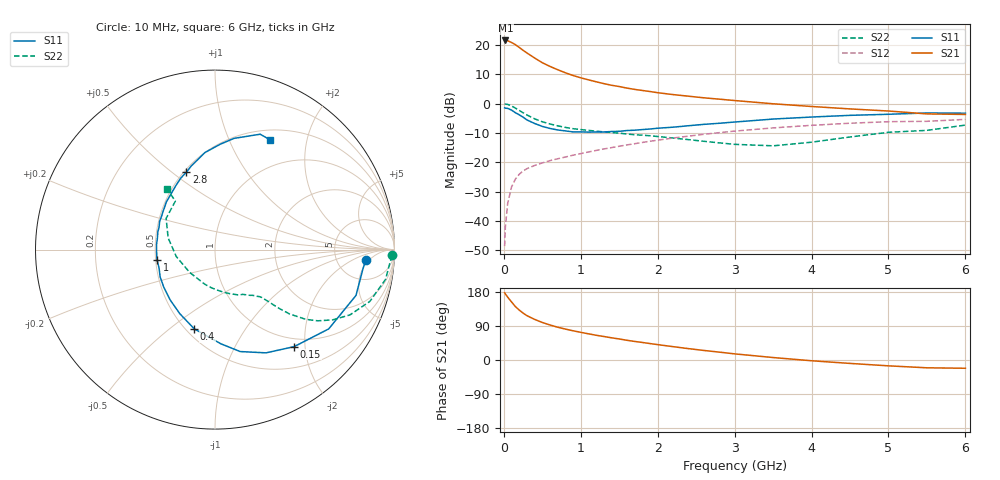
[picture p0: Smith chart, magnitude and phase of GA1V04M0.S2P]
! Infineon Technologies  Discrete & RF Semiconductors
! BF775
! Si NPN RF Bipolar Junction Transistor in SOT23
! VCE = 1 V  IC = 4 mA
! Common Emitter S-Parameters:  May  1996
# GHz  S  MA  R  50
!  f  S11  S21  S12  S22
! GHz  MAG  ANG  MAG  ANG  MAG  ANG  MAG  ANG
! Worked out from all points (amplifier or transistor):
!   36 points, 10 MHz to 6 GHz, reference 50 ohm
!   highest |S21| = 21.5 dB at 20 MHz (marker M1)
!   |S21| within 3 dB of that: start of sweep to 232.1 MHz
!   unconditionally stable (mu >= 1): 793.3 MHz to end of sweep
!   at 250 MHz: K = 0.44, MSG = 20.6 dB, |S12| = -23.0 dB
!   at 1.4 GHz: K = 1.17, MAG = 8.1 dB, |S12| = -15.0 dB
!   at 6 GHz: K = 1.04, MAG = -0.4 dB, |S12| = -5.4 dB
!   S11 on the Smith chart (normalised r, x): 10 MHz: 10, -4; 150 MHz: 0.85, -1.79; 400 MHz: 0.55, -0.61; 1 GHz: 0.51, -0.06; 2.8 GHz: 0.51, +0.56; 6 GHz: 0.62, +1.43
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0.01  0.8431 -3.8  11.81 177.4  0.0037 86.9  0.9891 -1.9
0.02  0.8318 -7.1  11.88 174.1  0.0079 85.2  0.9783 -4.0
0.05  0.826 -18.0  11.76 165.9  0.0198 79.5  0.9647 -9.9
0.1  0.7723 -34.9  10.98 153.3  0.0377 71.7  0.9096 -18.5
0.15  0.6977 -50.8  10.08 140.9  0.0515 64.3  0.8356 -25.8
0.2  0.6417 -63.7  9.053 131.9  0.0622 59.1  0.7628 -30.9
0.25  0.5852 -76.1  8.075 123.8  0.0707 55.3  0.6969 -34.7
0.3  0.5254 -86.5  7.28 117.0  0.0775 53.0  0.6386 -37.5
0.4  0.4564 -104.7  5.968 107.2  0.0879 49.8  0.5484 -40.8
0.5  0.4073 -118.8  4.961 99.0  0.0971 48.9  0.4888 -42.4
0.6  0.3756 -131.7  4.287 92.4  0.1063 48.4  0.4481 -43.4
0.7  0.3542 -143.5  3.769 86.5  0.1143 48.7  0.4164 -44.2
0.8  0.3415 -153.5  3.341 81.6  0.1224 48.7  0.3916 -45.0
1  0.3282 -170.2  2.743 73.0  0.14 49.6  0.3597 -46.7
1.1  0.3257 -178.0  2.533 69.1  0.1493 49.6  0.3489 -48.2
1.6  0.3464 152.9  1.831 52.0  0.1968 48.8  0.3021 -56.2
2.2  0.3949 128.4  1.42 35.2  0.2581 44.9  0.2582 -71.7
2.8  0.4605 110.2  1.187 20.8  0.3186 38.8  0.2134 -95.5
3.5  0.5437 95.9  0.99 6.5  0.3839 30.1  0.19 -138.1
4.5  0.6287 80.3  0.809 -9.0  0.4614 17.0  0.2691 166.0
5.5  0.6905 68.6  0.665 -20.6  0.4973 3.0  0.3487 129.3
6  0.6841 63.5  0.651 -21.8  0.5364 -0.9  0.4287 128.3
